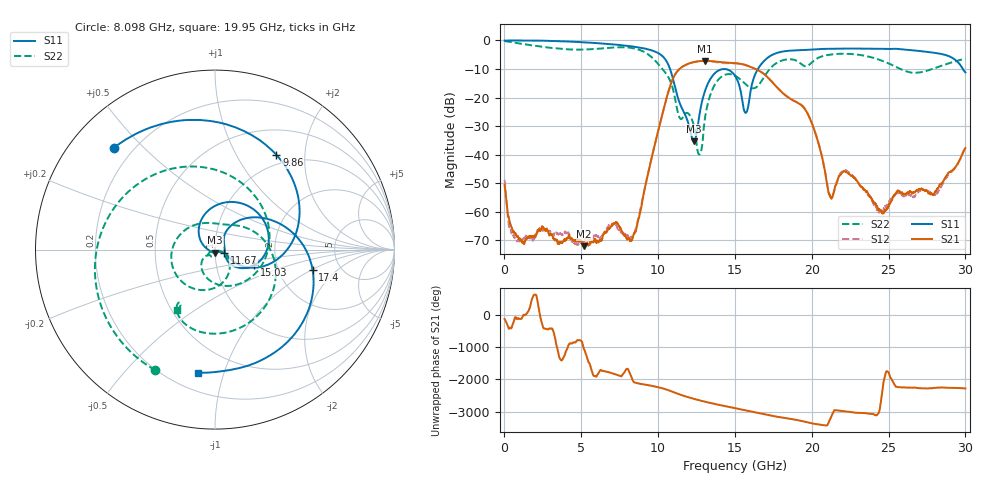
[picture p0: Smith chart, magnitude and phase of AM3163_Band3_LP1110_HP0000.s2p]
!Agilent Technologies,E8364B,MY43040894,A.07.50.67
!Agilent E8364B: A.07.50.67
!Date: Thursday, August 20, 2020 12:11:20
!Correction: S11(Full 2 Port(1,2))
!S21(Full 2 Port(1,2))
!S12(Full 2 Port(1,2))
!S22(Full 2 Port(1,2))
!S2P File: Measurements: S11, S21, S12, S22:
# Hz S  dB  R 50
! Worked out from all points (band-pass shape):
!   3201 points, 10 MHz to 30 GHz, reference 50 ohm
!   highest |S21| = -7.16 dB at 13.05 GHz (marker M1); lowest = -72.1 dB at 5.183 GHz (marker M2)
!   |S21| within 3 dB of the highest: 11.36 GHz to 16.4 GHz (5.044 GHz wide, 36.3 % of centre)
!   lowest |S11| = -35.3 dB at 12.32 GHz (marker M3), VSWR 1.04, Z = 50.1 - j1.72 ohm
!   |S11| at or under -10 dB: 10.78 GHz to 16.49 GHz (5.719 GHz wide, 41.9 % of centre); 29.83 GHz to end of sweep
!   |S22| runs from -40.0 to -0.2 dB; largest |S21 - S12| = 0.014
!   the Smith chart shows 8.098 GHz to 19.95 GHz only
!   S11 on the Smith chart (normalised r, x): 8.098 GHz: 0.13, +0.41; 9.86 GHz: 0.85, +1.48; 11.67 GHz: 1.11, -0.04; 15.03 GHz: 1.52, -0.28; 17.4 GHz: 3.13, -1.03; 19.95 GHz: 0.31, -0.82
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1e7  -0.04 -1.9  -50.64 -141.1  -48.80 -174.4  -0.20 -5.5
7.128906e8  -0.01 -19.5  -67.59 -78.6  -69.26 -161.5  -0.83 -51.0
2.606009e9  -0.10 -71.4  -66.24 -74.4  -66.35 40.4  -2.33 -164.3
5.014581e9  -0.60 -135.6  -70.33 -99.5  -70.96 152.6  -3.21 67.8
5.183275e9  -0.66 -140.1  -72.10 1.3  -70.63 -32.8  -3.19 58.6
6.579684e9  -1.15 -178.4  -67.14 40.9  -67.13 23.1  -2.69 -21.0
8.097928e9  -1.95 134.6  -69.29 49.2  -68.86 -12.7  -2.50 -116.3
9.859841e9  -4.02 57.1  -34.84 -71.4  -34.90 -71.6  -7.36 82.4
1.000979e10  -4.43 47.6  -31.56 -87.4  -31.63 -87.7  -8.27 60.8
1.166861e10  -25.06 -19.1  -8.92 6.5  -8.95 6.8  -26.40 -119.3
1.232464e10  -35.28 -86.8  -7.58 -85.8  -7.58 -85.6  -29.80 -154.1
1.304628e10  -17.79 134.6  -7.16 -174.3  -7.17 -174.8  -27.41 -18.1
1.5005e10  -12.38 -20.0  -7.97 -14.3  -7.97 -12.4  -12.33 -176.7
1.503312e10  -12.62 -22.0  -7.98 -17.0  -7.98 -15.2  -12.42 -179.2
1.571726e10  -25.33 9.7  -8.67 -85.2  -8.59 -84.6  -15.44 121.6
1.74042e10  -5.11 -11.8  -14.46 108.5  -14.42 109.2  -9.20 -14.6
1.995335e10  -3.18 -98.1  -28.32 -118.0  -28.18 -117.5  -7.97 -122.2
2.000958e10  -3.16 -99.5  -29.07 -123.7  -28.97 -123.2  -7.69 -123.1
2.12373e10  -2.92 -129.3  -55.09 50.1  -54.76 -176.6  -4.94 -164.8
2.500479e10  -2.98 144.1  -57.79 4.8  -56.66 -45.9  -8.07 40.9
2.714158e10  -3.78 83.9  -51.95 -119.8  -52.11 -110.0  -11.10 -101.1
3e10  -11.20 -31.4  -37.73 -124.8  -38.07 -125.1  -6.40 124.5
